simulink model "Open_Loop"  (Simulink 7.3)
settings: Solver=ode45  StartTime=0.0  StopTime=200  RelTol=1e-3
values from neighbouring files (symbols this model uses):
  J = [1045.3,  0,       19;      0,       641.02,  40;      19,      40,      505.05]    [run.m]    (also in start.m = [1.410986E+4, -0.3103E+2, -0.1187E+2;     -0.3103E+2,  1.304)
  npv = 28    [run.m]    (also in freq.m = 61)
undefined symbols (not defined in the file or in its folder): Au, Bu, Cu, Du

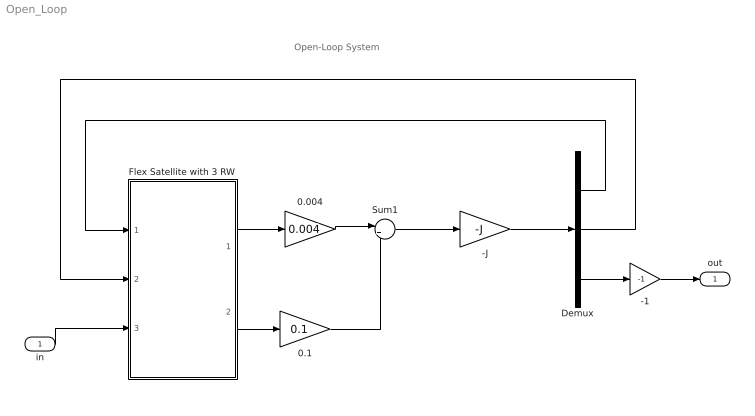
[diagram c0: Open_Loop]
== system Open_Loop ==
  note: Open-Loop System
  in : Inport  OutDataType=sfix(16)  OutScaling=2^0
  -1 : Gain  Gain=-1  ParameterDataType=sfix(16)  ParameterScaling=2^0  OutDataType=sfix(16)  OutScaling=2^0
  -J : Gain  Gain=-J  Multiplication=Matrix(K*u)  ParameterDataType=sfix(16)  ParameterScaling=2^0  OutDataType=sfix(16)  OutScaling=2^0
  0.004 : Gain  Gain=0.004  ParameterDataType=sfix(16)  ParameterScaling=2^0  OutDataType=sfix(16)  OutScaling=2^0
  0.1 : Gain  Gain=0.1  ParameterDataType=sfix(16)  ParameterScaling=2^0  OutDataType=sfix(16)  OutScaling=2^0
  Demux : Demux  Outputs=3
  Flex Satellite with 3 RW : Subsystem
  Sum1 : Sum  Inputs=|++  OutDataType=sfix(16)  OutScaling=2^0
  out : Outport  OutDataType=sfix(16)  OutScaling=2^0
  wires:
  Flex Satellite with 3 RW/2(rate) -> 0.1/1
  0.1/1 -> Sum1/2
  0.004/1 -> Sum1/1
  Flex Satellite with 3 RW/1(attit) -> 0.004/1
  Sum1/1 -> -J/1
  -J/1 -> Demux/1
  -1/1 -> out/1
  Demux/2 -> Flex Satellite with 3 RW/2(Ty)
  Demux/3 -> -1/1
  in/1 -> Flex Satellite with 3 RW/3(Tz)
  Demux/1 -> Flex Satellite with 3 RW/1(Tx)

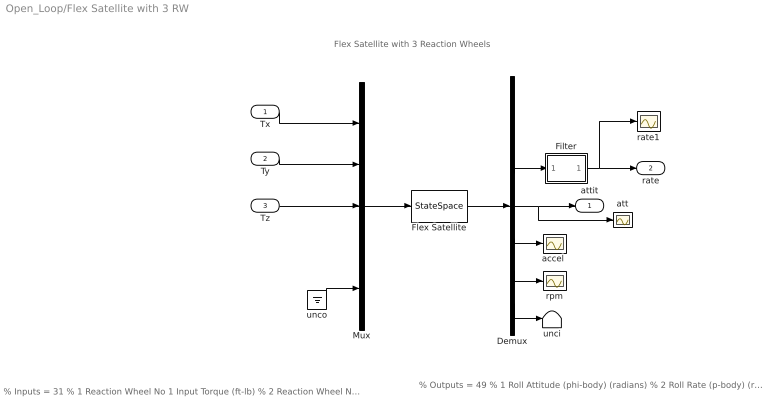
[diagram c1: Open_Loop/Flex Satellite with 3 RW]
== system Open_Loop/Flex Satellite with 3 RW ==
  note: Flex Satellite with 3 Reaction Wheels
  note: % Outputs = 49 % 1 Roll Attitude (phi-body) (radians) % 2 Roll Rate (p-body) (rad/sec) % 3 Pitch Attitude (thet-bdy) (radians) % 4 Pitch Rate (q-body) (rad/sec) % 5 Yaw Attitude (psi-body) (radians) % 6 Yaw Rate (r-body) (rad/sec) % 7 Angle of attack, alfa, (radians) % 8 Angle of sideslip, beta, (radian) % 9 Change in Altitude, delta-h, (feet) % 10 Forward Acceleration (V-dot) (ft/sec) % 11 Cross Range Velocity (Vcr) (ft/sec) % 12 Rate-Gyro # 1, Roll Rate (Body) (rad/sec) % 13 Rate-Gyro # 2, Pitch Rate (Body) (rad/sec) % 14 Rate-Gyro # 3, Yaw Rate (Body) (rad/sec) % 15 Gyro # 4, Roll Attitude (Body) (radians) % 16 Gyro # 5, Pitch Attitude (Body) (radians) % 17 Gyro # 6, Yaw Attitude (Body) (radians) % 18 Accelerom # 1, (along X), (ft/sec^2) Translat. Acceler % 19 Accelerom # 2, (along Y), (ft/sec^2) Translat. Acceler % 20 Reaction Wheel # 1 Rate (rpm) relative to vehicle % 21 Reaction Wheel # 2 Rate (rpm) relative to vehicle % 22 Reaction Wheel # 3 Rate (rpm) relative to vehicle
  note: % Inputs = 31 % 1 Reaction Wheel No 1 Input Torque (ft-lb) % 2 Reaction Wheel No 2 Input Torque (ft-lb) % 3 Reaction Wheel No 3 Input Torque (ft-lb) % 4 Ext Torque Direct.=( 0.0000 1.0000 0.0000)
  Tx : Inport  OutDataType=sfix(16)  OutScaling=2^0
  Ty : Inport  Port=2  OutDataType=sfix(16)  OutScaling=2^0
  Tz : Inport  Port=3  OutDataType=sfix(16)  OutScaling=2^0
  Demux : Demux  Outputs="[6, 5, 3, 3, 2, 3,  npv]"
  Filter : Subsystem
  Flex Satellite : StateSpace  A=Au  B=Bu  C=Cu  D=Du
  Mux : Mux  Inputs="[1,1,1, 1,  npv]"
  "accel " : Scope
  att : Scope
  rate1 : Scope
  rpm : Scope
  unci : Terminator
  unco : Ground
  attit : Outport  OutDataType=sfix(16)  OutScaling=2^0
  rate : Outport  Port=2  OutDataType=sfix(16)  OutScaling=2^0
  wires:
  Demux/4 -> attit/1, att/1
  Demux/3 -> Filter/1(In)
  Demux/5 -> "accel "/1
  Demux/6 -> rpm/1
  Mux/1 -> Flex Satellite/1
  Flex Satellite/1 -> Demux/1
  Tx/1 -> Mux/1
  Tz/1 -> Mux/3
  Ty/1 -> Mux/2
  Filter/1(Ou) -> rate/1, rate1/1
  unco/1 -> Mux/5
  Demux/7 -> unci/1

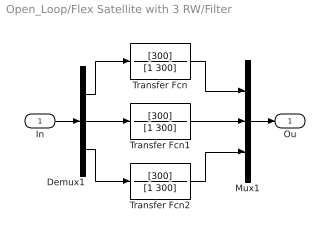
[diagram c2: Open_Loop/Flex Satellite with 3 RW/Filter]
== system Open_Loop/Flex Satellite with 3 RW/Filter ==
  In : Inport  OutDataType=sfix(16)  OutScaling=2^0
  Demux1 : Demux  Outputs=3
  Mux1 : Mux  Inputs=3
  Transfer Fcn : TransferFcn  Numerator=[300]  Denominator=[1 300]
  Transfer Fcn1 : TransferFcn  Numerator=[300]  Denominator=[1 300]
  Transfer Fcn2 : TransferFcn  Numerator=[300]  Denominator=[1 300]
  Ou : Outport  OutDataType=sfix(16)  OutScaling=2^0
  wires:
  Transfer Fcn1/1 -> Mux1/2
  Transfer Fcn/1 -> Mux1/1
  Transfer Fcn2/1 -> Mux1/3
  Demux1/2 -> Transfer Fcn1/1
  Demux1/1 -> Transfer Fcn/1
  Demux1/3 -> Transfer Fcn2/1
  In/1 -> Demux1/1
  Mux1/1 -> Ou/1
